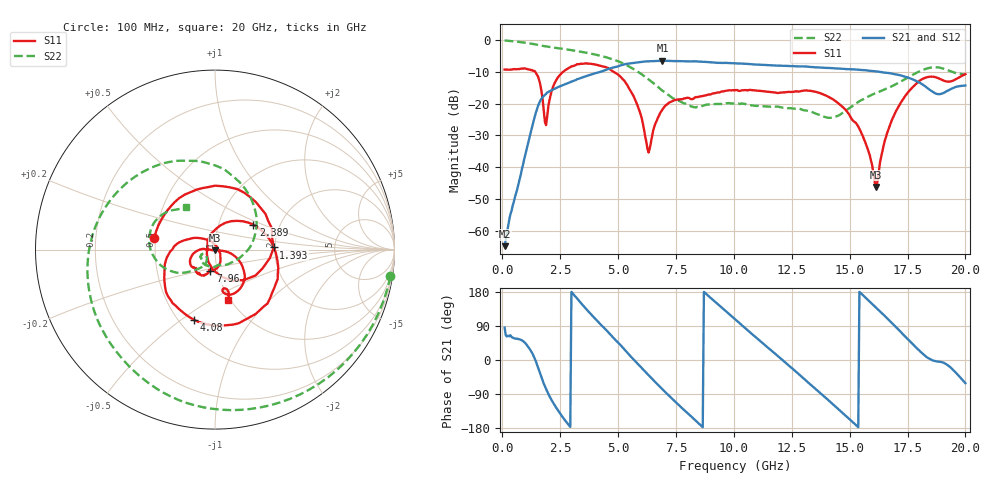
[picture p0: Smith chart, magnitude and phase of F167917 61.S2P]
!  2-Port S-parameters saved by WinCal
! VAR MeasName=S-Parameters (CALIBRATED_DATA) read from VNA (N5242A)
! VAR MeasDate=2016-11-22 9:03:02
! VAR NAME=F167917 61
! VAR FILENAME=F167917 61.S2P
! VAR DATE=2016-11-22 9:03:02
! VAR PHYS_PORTS=1,2
# Hz S DB R 50
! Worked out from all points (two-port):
!   401 points, 100 MHz to 20 GHz, reference 50 ohm
!   highest |S21| = -6.50 dB at 6.916 GHz (marker M1); lowest = -64.9 dB at 100 MHz (marker M2)
!   |S21| within 3 dB of the highest: 4.422 GHz to 15.69 GHz (11.27 GHz wide, 112 % of centre)
!   lowest |S11| = -46.2 dB at 16.12 GHz (marker M3), VSWR 1.01, Z = 49.8 - j0.452 ohm
!   |S11| at or under -10 dB: 1.425 GHz to 2.624 GHz (1.199 GHz wide, 59.2 % of centre); 4.813 GHz to end of sweep
!   |S22| runs from -24.5 to -0.1 dB; largest |S21 - S12| = 0.0041
!   S11 on the Smith chart (normalised r, x): 100 MHz: 0.49, +0.07; 1.393 GHz: 1.97, +0.05; 2.389 GHz: 1.47, +0.44; 4.08 GHz: 0.60, -0.56; 7.96 GHz: 0.92, -0.22; 20 GHz: 0.97, -0.60
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1e8  -9.27 168.7  -64.92 85.6  -65.11 83.3  -0.10 -8.7
8.4625e8  -8.98 82.4  -40.64 51.9  -40.68 52.0  -0.67 -66.9
1.3935e9  -9.70 2.1  -24.30 5.0  -24.34 5.3  -1.29 -103.7
1.64225e9  -14.03 -60.8  -19.03 -37.2  -19.03 -36.9  -1.66 -118.4
1.891e9  -26.77 154.8  -16.92 -75.9  -16.91 -75.7  -1.99 -131.5
2.3885e9  -11.86 33.0  -14.85 -131.4  -14.86 -131.3  -2.50 -155.8
3.43325e9  -7.46 -61.5  -11.81 147.6  -11.76 147.9  -3.70 158.3
4.08e9  -7.78 -106.5  -10.30 104.4  -10.22 104.5  -4.64 131.0
5.3735e9  -13.87 168.4  -7.46 21.2  -7.44 20.9  -7.92 70.5
6.31875e9  -35.42 24.4  -6.67 -40.3  -6.67 -40.4  -12.39 21.2
6.7665e9  -23.82 -61.9  -6.51 -67.9  -6.52 -68.0  -15.04 -3.0
6.91575e9  -21.86 -70.0  -6.50 -77.2  -6.51 -77.3  -15.93 -10.1
7.9605e9  -18.21 -102.3  -6.68 -137.9  -6.65 -138.0  -20.18 -63.3
8.90575e9  -17.16 -107.4  -6.92 168.8  -6.91 168.8  -20.25 -95.7
1.005e10  -15.79 -121.1  -7.32 107.7  -7.31 107.7  -19.94 -130.3
1.179125e10  -16.52 -136.0  -8.00 16.0  -7.96 15.9  -20.97 -152.6
1.338325e10  -16.09 -152.0  -8.46 -68.7  -8.43 -68.7  -22.68 -161.1
1.53235e10  -26.64 178.0  -9.28 -174.6  -9.29 -174.8  -19.70 -124.7
1.61195e10  -46.25 -111.3  -9.82 139.7  -9.88 139.7  -16.74 -131.7
1.67165e10  -27.22 -9.0  -10.39 104.4  -10.45 104.6  -14.89 -137.9
1.805975e10  -12.60 -46.0  -13.54 21.8  -13.48 22.4  -9.71 -167.8
2e10  -10.70 -75.9  -14.29 -61.1  -14.16 -61.0  -10.86 124.3
